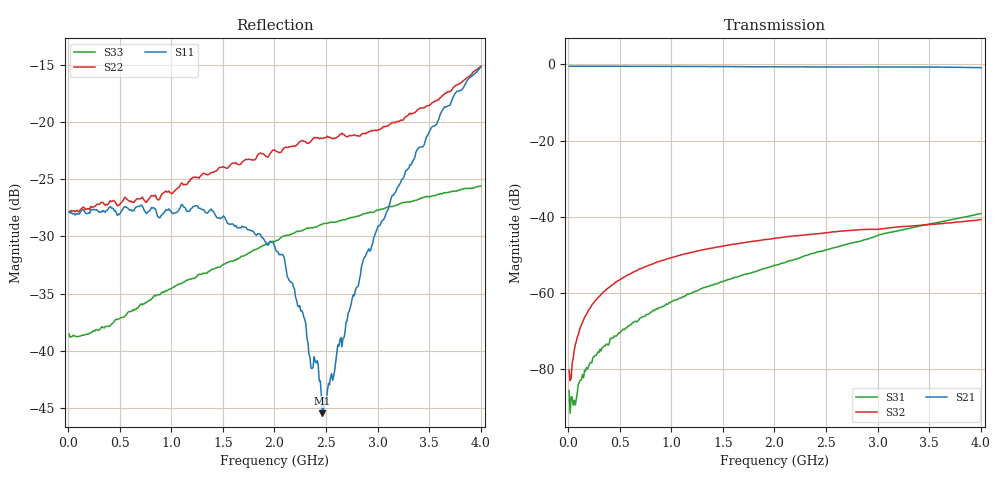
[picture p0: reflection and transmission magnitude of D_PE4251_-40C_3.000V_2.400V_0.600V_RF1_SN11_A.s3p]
! Device ID: PE4251_SoldCshunt_081809
! Dir: c:\Test Bench Repositories\Bench_Software_CVI_Version_8\trunk\PSC 4Port_VNA Bench\datalog\4250\TEST\PE4251_SoldCshunt_081809\-40C\3p000000\RF1
! Serial: 11
! Insertion: A
! Temp: -40C
! VDD: 3.000
! Control_Hi: 80.000
! Control_Lo: 20.000
! Logic State: RF1
! Port 1: RFC
! Port 2: RF1
! Port 3: RF2
! V1 = 0.60
! V2 = 2.40
! V3 = 0.60
! IDD: 4.793110e-05
! FILE NAME
! DATE 08/18/09  20:08
! CORRECTED  DATA
#  Hz  S  RI  R  50.00
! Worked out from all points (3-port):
!   401 points, 10 MHz to 4 GHz, reference 50 ohm
!   strongest paths, dB at 10 MHz, 1.008 GHz, 2.005 GHz, 3.002 GHz, 4 GHz:
!     S21: -0.5, -0.5, -0.6, -0.7, -0.9
!     S32: -80.2, -50.6, -45.6, -43.3, -40.7
!     S31: -85.6, -62.2, -52.7, -44.8, -39.2
!   lowest |S11| = -45.5 dB at 2.464 GHz (marker M1), VSWR 1.01, Z = 50.1 - j0.524 ohm
!   |S11| at or under -10 dB: start of sweep to end of sweep
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1e7  0.0405 0.000385  0.9445 -0.00325  2.87e-05 -0.000136
     0.9446 -0.00419  0.0407 0.000212  7.49e-05 -3.03e-05
     4.23e-05 -3.14e-05  5.23e-05 -8.26e-05  0.0118 -0.000294
1.79575e8  0.0398 0.000852  0.943 -0.061  -1.32e-05 -9.82e-05
           0.9426 -0.0608  0.0417 0.000498  4.27e-05 0.000547
           -1.52e-05 -0.000105  4.42e-05 0.000531  0.0117 0.00164
4.78825e8  0.039 -0.00307  0.9292 -0.1591  -0.000149 -0.000251
           0.9286 -0.1589  0.0429 -0.00341  0.000139 0.00142
           -0.00014 -0.000248  0.000142 0.00144  0.0131 0.00398
1.157125e9  0.0387 -0.0124  0.862 -0.3684  -0.000847 -0.000437
            0.8625 -0.3676  0.0519 -0.0143  0.000625 0.00327
            -0.000861 -0.000442  0.000621 0.00326  0.0166 0.0117
2.005e9  0.0265 -0.0101  0.723 -0.5818  -0.00227 -0.000463
         0.7227 -0.5821  0.0669 -0.035  0.0012 0.00508
         -0.00227 -0.00046  0.0012 0.00509  0.0181 0.024
2.2843e9  0.0103 -0.00956  0.6679 -0.6419  -0.003 -0.000551
          0.6666 -0.6427  0.0645 -0.0516  0.00137 0.00559
          -0.00301 -0.000554  0.00136 0.0056  0.0166 0.0295
2.46385e9  0.000953 -0.00523  0.6311 -0.6768  -0.00352 -0.000497
           0.6297 -0.6764  0.0616 -0.0583  0.00136 0.00594
           -0.00351 -0.000518  0.00135 0.00595  0.0151 0.0324
2.86285e9  -0.018 -0.0176  0.539 -0.7535  -0.00493 -0.000446
           0.5396 -0.7511  0.0429 -0.0783  0.00149 0.00664
           -0.00495 -0.000449  0.00149 0.00667  0.0106 0.0383
3.14215e9  -0.0366 -0.0307  0.4678 -0.7982  -0.00635 -4.03e-05
           0.4685 -0.7968  0.0224 -0.0969  0.00115 0.00715
           -0.00635 -4.81e-05  0.00114 0.00717  0.00635 0.0423
4e9  -0.1565 -0.0777  0.1883 -0.8877  -0.0108 0.0021
     0.1875 -0.8852  -0.1195 -0.1294  -4.9e-06 0.0092
     -0.0108 0.00207  -2.68e-05 0.00921  -0.0142 0.0506
